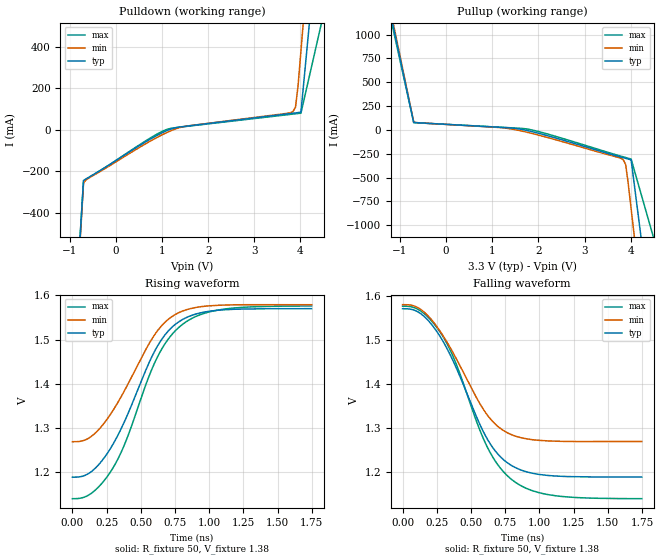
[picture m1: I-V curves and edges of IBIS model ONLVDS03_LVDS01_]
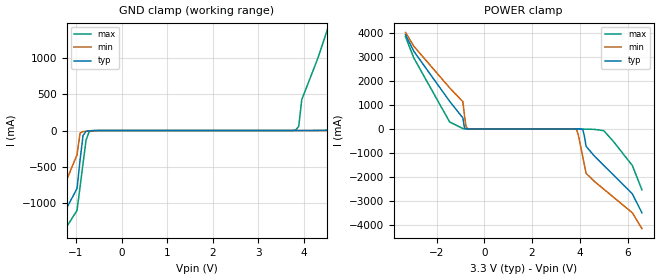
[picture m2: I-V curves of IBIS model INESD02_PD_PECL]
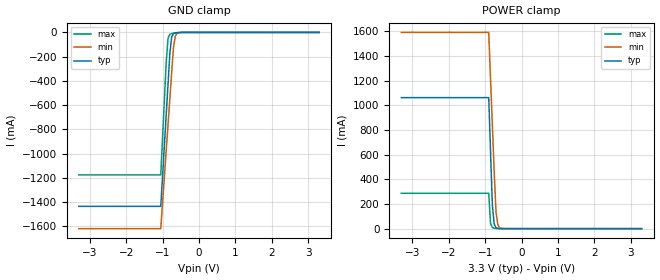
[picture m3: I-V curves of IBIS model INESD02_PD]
|   This file is an IBIS representation of the   |
|   Integrated Device Technology, Inc.   |
|   ICS8741004   |
|   DIFFERENTIAL-TO-LVDS/0.7V DIFFERENTIAL PCI EXPRESS JITTER ATTENUATOR   |
[IBIS Ver]   4.1
[File name]   8741004_3v3.ibs
[File Rev]   0.0
[Date]   13 Jul 2009 | Last modified
|   May 22 2006 | Generated
[Source]   Originated at Integrated Device Technology, Inc.
[Disclaimer]
IDT hereby grants the user of this IBIS model a non-exclusive,
nontransferable license to use this IBIS model under the following terms.
Before using this IBIS model, the user should read this license.
If the user does not accept these terms,  the IBIS model should be
returned to IDT within 30 days.
   The user is granted this license only to use the IBIS model and
is not granted rights to sell, load, rent, lease or license the IBIS
model in whole or in part, or in modified form to anyone other than
user. User may modify the IBIS model to suit its specific
applications but rights to derivative works and such modifications
shall belong to IDT.
   This IBIS model is provided on an "AS IS" basis and IDT makes
absolutely no warranty with respect to the information contained
herein. IDT DISCLAIMS AND CUSTOMER WAIVES ALL WARRANTIES, EXPRESS
OR IMPLIED, INCLUDING WARRANTIES OF MERCHANTABILITY OR FITNESS FOR
A PARTICULAR PURPOSE. The entire risk as to quality and performance
is with the Customer. ACCORDINGLY, IN NO EVENT SHALL THE COMPANY BE
LIABLE FOR ANY DAMAGES, WHETHER IN CONTRACT OR TORT,INCLUDING ANY
LOST PROFITS OR OTHER INCIDENTAL, CONSEQUENTIAL, EXEMPLARY, OR
PUNITIVE DAMAGES ARISING OUT OF THE USE OR APPLICATION OF THE IBIS
model provided in this package. Further, IDT reserves the right to
make changes without notice to any product herein to improve
reliability, function, or design. IDT does not convey any license
under patent rights or any other intellectual property rights,
including those of third parties.
   IDT is not obligated to provide maintenance or support
for the licensed IBIS model.
[Copyright]   Copyright 2006 by Integrated Device Technology, Inc.
[Component]   ICS8741004AG
[Manufacturer] Integrated Device Technology, Inc.
[Package]
|TSSOP 24 Lead
|   typ   min   max
R_pkg   60.65m   52.4m   68.9m
L_pkg   1.989nH   1.431nH   2.547nH
C_pkg   0.314pF   0.254pF   0.374pF
[Pin] signal_name  model_name   R_pin   L_pin   C_pin
1   nQA1   ONLVDS03_LVDS01_   68.9m   2.547n   0.374p
2   QA1   ONLVDS03_LVDS01_   65.6m   2.323n   0.350p
3   VDDO   POWER   62.3m   2.100n   0.326p
4   QA0   ONLVDS03_LVDS01_   59.0m   1.877n   0.302p
5   nQA0   ONLVDS03_LVDS01_   55.7m   1.654n   0.278p
6   MR   INESD02_PD_PECL   52.4m   1.431n   0.254p
7   BW_SEL   NC   52.4m   1.431n   0.254p
8   nc   NC   55.7m   1.654n   0.278p
9   VDDA   POWER   59.0m   1.877n   0.302p
10   F_SELA   INESD02_PD   62.3m   2.100n   0.326p
11   VDD   POWER   65.6m   2.323n   0.350p
12   OEA   INESD02_PU   68.9m   2.547n   0.374p
13   CLK   INESD02_PD_PECL   68.9m   2.547n   0.374p
14   nCLK   INESD02_PU_PECL   65.6m   2.323n   0.350p
15   GND   GND   62.3m   2.100n   0.326p
16   GND   GND   59.0m   1.877n   0.302p
17   OEB   INESD02_PU   55.7m   1.654n   0.278p
18   F_SELB   INESD02_PD   52.4m   1.431n   0.254p
19   IREF   NC   52.4m   1.431n   0.254p
20   nQB0   DCMOUT01_ISO_VRE   55.7m   1.654n   0.278p
21   QB0   DCMOUT01_ISO_VRE   59.0m   1.877n   0.302p
22   VDDO   POWER   62.3m   2.100n   0.326p
23   QB1   DCMOUT01_ISO_VRE   65.6m   2.323n   0.350p
24   nQB1   DCMOUT01_ISO_VRE   68.9m   2.547n   0.374p
[Diff Pin]  inv_pin  vdiff tdelay_typ tdelay_min  tdelay_max
|Outputs
1   2   NA   0   0   0
4   5   NA   0   0   0
21   20   NA   0   0   0
23   24   NA   0   0   0
|Input
13   14   0.15   0   0   0
| Models and submodels in the file (6): ONLVDS03_LVDS01_ (Output), INESD02_PD_PECL (Input), INESD02_PD (Input), INESD02_PU (Input), INESD02_PU_PECL (Input), DCMOUT01_ISO_VRE (Open_source)
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[Model]   ONLVDS03_LVDS01_
Model_type   Output
Polarity   Non-Inverting
|   typ   min   max
C_comp   2pF   1.5pF   2.5pF
Vmeas = 1.38V
Rref = 50
Cref = 0
Vref = 1.38V
|   typ   min   max
[Voltage range]   3.3V   3.135V   3.465V
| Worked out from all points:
|   slope of the pulldown table from 0 to 0.495 V, typ, clamps not added: 7.07 ohm
|   slope of the pullup table from 0 to 0.495 V, typ, clamps not added: 37.1 ohm
|   rising waveform, R_fixture 50, V_fixture 1.38: 20-80 % time 338ps typ, 336ps min, 345ps max; typ from 1.19 V to 1.57 V
|   falling waveform, R_fixture 50, V_fixture 1.38: 20-80 % time 338ps typ, 336ps min, 345ps max; typ from 1.57 V to 1.19 V
[Pulldown]
|Voltage   I (typ)   I (min)   I (max)
-3.3V     -12.71A    -11.01A    -15.57A
-1.22V    -2.163A    -2.22A     -2.109A
-700mV    -243.4mA   -255.4mA   -245.9mA
-591mV    -228.8mA   -232.9mA   -231.1mA
975.4mV   -17.01mA   -26.96mA   -10.67mA
1.461V    15.81mA    15.11mA    14.81mA
3.838V    79.93mA    87.99mA    75.84mA
3.892V    81.43mA    109mA      77.23mA
3.946V    83mA       208.7mA    78.62mA
4.01V     85.14mA    379.8mA    80.26mA
4.528V    1.294A     1.77A      585mA
6.6V      7.984A     7.36A      9.101A
[Pullup]
|Voltage   I (typ)   I (min)   I (max)
-3.3V     7.976A     6.908A     9.771A
-1.22V    1.261A     1.299A     1.219A
-700mV    77.14mA    81.31mA    75.55mA
1.191V    25.7mA     22.95mA    26.95mA
1.732V    -4.369mA   -22.72mA   10.36mA
3.784V    -284.8mA   -297.7mA   -275.6mA
3.838V    -291.9mA   -312.5mA   -283.1mA
3.892V    -299mA     -365.3mA   -290.5mA
3.946V    -306.1mA   -559.4mA   -297.8mA
4.01V     -314.8mA   -828mA     -306.5mA
4.528V    -2.273A    -3.003A    -1.186A
6.6V      -12.73A    -11.74A    -14.49A
[Ramp]
|   typ   min   max
dV/dt_r   0.305/0.523n   0.248/0.506n   0.349/0.557n
dV/dt_f   0.305/0.523n   0.248/0.506n   0.349/0.557n
R_load =   50.0000
[Rising Waveform]
R_fixture = 50
V_fixture = 1.38   |Vcc_typ
V_fixture_min = 1.38 |Vcc_min
V_fixture_max = 1.38 |Vcc_max
C_fixture = 0.0p
| Time   typ   min   max
0s        1.188V     1.268V     1.139V
140.1ps   1.201V     1.281V     1.152V
287.3ps   1.258V     1.335V     1.204V
387.1ps   1.319V     1.388V     1.267V
613.1ps   1.481V     1.516V     1.455V
700.7ps   1.519V     1.546V     1.501V
797ps     1.544V     1.564V     1.533V
924.9ps   1.56V      1.574V     1.555V
1.09ns    1.567V     1.578V     1.568V
1.748ns   1.57V      1.579V     1.576V
[Falling Waveform]
R_fixture = 50
V_fixture = 1.38   |Vcc_typ
V_fixture_min = 1.38 |Vcc_min
V_fixture_max = 1.38 |Vcc_max
C_fixture = 0.0p
| Time   typ   min   max
0s        1.571V     1.58V      1.576V
140.1ps   1.558V     1.567V     1.564V
287.3ps   1.501V     1.513V     1.511V
387.1ps   1.44V      1.46V      1.449V
613.1ps   1.278V     1.332V     1.26V
700.7ps   1.239V     1.302V     1.214V
797ps     1.215V     1.285V     1.183V
924.9ps   1.199V     1.274V     1.16V
1.09ns    1.192V     1.27V      1.147V
1.748ns   1.189V     1.269V     1.139V
[Model]   INESD02_PD_PECL
Model_type  Input
Polarity   Non-Inverting
Vinl = 0.8V
Vinh = 2.0V
|   typ   min   max
C_comp   2pF   1.5pF   2.5pF
|   typ   min   max
[Voltage range]  3.3V   3.15V   3.45V
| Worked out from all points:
|   GND clamp passes 1 mA (typ) near -0.59 V on its own axis
|   POWER clamp passes 1 mA (typ) near -0.70 V on its own axis
[GND_clamp]
-3.3V     -3.894A    -4.294A    -3.674A
-1.6V     -1.569A    -1.322A    -1.74A
-974.8mV  -794.1mA   -331.5mA   -1.096A
-843.4mV  -68.33mA   -15.34mA   -452.9mA
-646.5mV  -1.912mA   -4.151mA   -2.665mA
3.818V    89.38uA    70.49uA    7.198mA
3.95V     342.2uA    75.94uA    423.8mA
4.6V      7.437mA    165.5uA    1.553A
4.9V      78.32mA    440.9uA    2.118A
5.5V      1.293A     2.769mA    3.249A
6.25V     2.651A     112.4mA    4.38A
6.6V      3.331A     896.1mA    4.946A
[POWER_clamp]
-3.3V     3.923A     4.017A     3.838A
-2.95V    3.23A      3.44A      2.951A
-1.45V    1.149A     1.709A     289.6mA
-896.9mV  456.5mA    1.133A     15.4mA
-762.9mV  4.223mA    91.07mA    1.486mA
-695.9mV  792.2uA    10.73mA    555.6uA
3.861V    -556.7uA   -26.14mA   -39.45uA
4.129V    -41.85mA   -1.19A     -4.904mA
4.263V    -724.2mA   -1.847A    -12.04mA
5V        -1.514A    -2.505A    -71.38mA
6.2V      -2.701A    -3.492A    -1.525A
6.6V      -3.492A    -4.151A    -2.536A
[Model]   INESD02_PD
Model_type   Input
Polarity   Non-Inverting
Vinl = 0.80V
Vinh = 2.0V
|   typ   min   max
C_comp   2pF   1.5pF   2.5pF
|   typ   min   max
[Voltage range]  3.3V   3.15V   3.45V
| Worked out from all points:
|   GND clamp passes 1 mA (typ) near -0.56 V on its own axis
|   POWER clamp passes 1 mA (typ) near -0.61 V on its own axis
[GND_clamp]
|Voltage   I(typ)   I(min)   I(max)
-3.3V     -1.436A    -1.62A     -1.176A
-1.05V    -1.436A    -1.62A     -1.176A
-900mV    -678.5mA   -975.1mA   -244mA
-850mV    -426.1mA   -760.1mA   -46.85mA
-800mV    -173.9mA   -545.4mA   -16.11mA
-750mV    -36.96mA   -330.7mA   -9.916mA
-700mV    -9.696mA   -120.2mA   -7.056mA
-650mV    -3.545mA   -29.7mA    -4.857mA
-600mV    -1.629mA   -7.52mA    -3.049mA
-400mV    -52.81uA   -52.52uA   -108.7uA
3.3V      71.13uA    77.43uA    62.11uA
[POWER_clamp]
|Voltage   I(typ)   I(min)   I(max)
-3.3V     1.063A     1.593A     287.3mA
-900mV    1.063A     1.593A     287.3mA
-850mV    620.5mA    1.215A     41.84mA
-800mV    191.6mA    837.5mA    8.757mA
-750mV    37.76mA    460.2mA    3.328mA
-700mV    8.104mA    133.8mA    1.728mA
-650mV    2.076mA    32.66mA    905.3uA
-600mV    678.1uA    8.083mA    443.8uA
-450mV    104.2uA    213.3uA    89.09uA
3.3V      -3.041nA   -3.986uA   0A
